(* Logix 5000 Rung export; software revision 16.04 *)

MODULES
   Local : vendor None type None code None
   GSC : vendor None type None code None
END_MODULES

TYPE GSCBLOCKSTATUS :   // This shows all blocks that were used by the module
STRUCT
   Read : INT;   // Number of blocks read by the module
   Write : INT;   // Number of blocks written by the module
   Parse : INT;   // Number of blocks parsed by the module
   Err : INT;   // Number of block transfer errors
END_STRUCT
END_TYPE

TYPE GSCCONTROL :   // Ladder send special blocks to request the module to perform the request
STRUCT
   Warmboot : BOOL;   // Performs a warm boot operation on the module (software reset).
   Coldboot : BOOL;   // Performs a cold boot operation on the module (hardware and software reset).
   ConfigDone : BOOL;   // Confirms the module received its configuration from ladder logic
END_STRUCT
END_TYPE

TYPE GSCPORTDATA :   // Individual port data
STRUCT
   ReadLength : INT;   // The length of character the port is rescieving
   ReadString : SINT[4096];   // Where received data will be displayed
   WriteLength : INT;   // The length of character the port is transmitting
   WDelay : INT;   // Number of milliseconds to wait between each character sent from the port
   WriteString : SINT[4096];   // Where sent data will be placed before it is sent
END_STRUCT
END_TYPE

TYPE GSCERRORWORD :   // Bit coded error word for configuration and overflow error for MVI56-GSC module.
STRUCT
   Cfg_type : BOOL;   // Bit 0, type field configuration error
   Cfg_Baud : BOOL;   // Bit 1, baud rate field configuration error
   Cfg_Parity : BOOL;   // Bit 2, parity field configuration error
   Cfg_DataBits : BOOL;   // Bit 3, data bit field configuration error
   Cfg_StopBits : BOOL;   // Bit 4, stop bit field configuration error
   Cfg_Handshake : BOOL;   // Bit 5, handshaking field configuration error
   Cfg_RTermcount : BOOL;   // Bit 6, receive termination character count field configuration error
   Cfg_RPacketLen : BOOL;   // Bit 7, receive packet length field configuration error
   Cfg_RTimeout : BOOL;   // Bit 8, receive message timeout field configuration error
   Cfg_RDelay : BOOL;   // Bit 9, receive intercharacter delay field configuration error
   Cfg_WTimeout : BOOL;   // Bit 10, write message timeout field configuration error
   Resv_Bit11 : BOOL;   // Bit 11
   Resv_Bit12 : BOOL;   // Bit 12
   Resv_Bit13 : BOOL;   // Bit 13
   Resv_Bit14 : BOOL;   // Bit 14
   Err_ROverflow : BOOL;   // Bit 15, receive overflow error
END_STRUCT
END_TYPE

TYPE GSCPORTSTAT :   // Port status Data
STRUCT
   RxState : INT;   // State of receive task
   RxCharCnt : INT;   // Number of characters received on port
   RxMsgCnt : INT;   // Number of messages received on port
   TxState : INT;   // State of transmit task
   TxCharCnt : INT;   // Number of characters transmitted on port
   TxMsgCnt : INT;   // Number of messages transmitted on port
   ErrorWord : GSCERRORWORD;   // Error/Configuration Word for port
END_STRUCT
END_TYPE

TYPE GSCMODULEDEF :   // This defines the complete module tags
STRUCT
   CONFIG : GSCPORTCONFIG;   // Port configuration parameters
   DATA : GSCDATA;   // Port sent and received data
   STATUS : GSCSTATUS;   // Module status data and individual port status
   CONTROL : GSCCONTROL;   // Module control parameters
   UTIL : GSCUTIL;   // Tags used by the module
END_STRUCT
END_TYPE

TYPE GSCUTIL :   // Used by the module for block hand shaking
STRUCT
   LastRead : SINT;   // This is used to read the input image from the processor
   LastWrite : SINT;   // This is used to write the output image to the processor
   BackplaneFail : INT;   // This is used to control number of backplane failures before module stops communicating on both gsc ports
   P1WriteLast : INT;   // Port 1 last write data in the array
   P2Writelast : INT;   // Port 2 last data in the array
   P1ArrayIndex : INT;   // This is the index reference within the read or write data array for port1
   P2ArrayIndex : INT;   // This is the index reference within the read or write data array for port 2
   P1RSindex : INT;   // used when more than 200 characters are received on the port 1
   P2RSindex : INT;   // used when more than 200 characters are received on the port 2
   P1Temp1 : INT;   // This temp parameter for port 1 is used to copy SINT to an INT in order to read a vlaue is higher than 127 characters
   P2Temp2 : INT;   // This temp parameter for port 2 is used to copy SINT to an INT in order to read a vlaue is higher than 127 characters
   Scratch1 : INT;   // Used to calculate number of characters read by the port
   Scratch2 : INT;   // Used to calculate number of characters read by the port
END_STRUCT
END_TYPE

TYPE GSCDATA :   // The following contains the data read in on the port and to be written out the port.
STRUCT
   Port1 : GSCPORTDATA;   // Port 1 data
   Port2 : GSCPORTDATA;   // Port 2 data
END_STRUCT
END_TYPE

TYPE GSCPORTCONFIG :   // Shows both ports configuration
STRUCT
   Port1 : GSCPORTCONFIGPARA;   // Port 1 configuration data
   Port2 : GSCPORTCONFIGPARA;   // Port 2 configuration data
END_STRUCT
END_TYPE

TYPE GSCSTATUS :   // Module Status data
STRUCT
   PassCnt : INT;   // Program cycle counter for module
   Product : INT[2];   // Product code for module (GSC)
   Rev : INT[2];   // Revision level of module's code
   OP : INT[2];   // Operating system version for module
   Run : INT[2];   // Run number for module
   BlockStatus : GSCBLOCKSTATUS;   // Data block transfer statistics
   Port1 : GSCPORTSTAT;   // Status for port1
   Port2 : GSCPORTSTAT;   // Status for port 2
END_STRUCT
END_TYPE

TYPE GSCPORTCONFIGPARA :   // The following are the configuration parameters for the port of the MVI56-GSC module.
STRUCT
   Enabled : INT;   // 0=Disable port, 1=Enable port
   Type : INT;   // Type of control used to flush data received on port
   Baudrate : INT;   // Baud rate for communications
   Parity : INT;   // Parity (0=none, 1=odd, 2=even, 3=mark, 4=space)
   DataBits : INT;   // Data bits (5, 6, 7, or 8)
   StopBits : INT;   // Stop bits (1 or 2)
   RTSOn : INT;   // RTS delay before sending data
   RTSOff : INT;   // RTS delay after sending message
   Handshaking : INT;   // Type of Handshaking (0=none, 1=RTSCTS, 2=DTRDSR,3=XONXOFF)
   RTermCnt : INT;   // Number of termination characters for received message for control
   RTermChar : SINT[12];   // Characters for termination control
   RPacketLen : INT;   // Fixed packet length value
   RTimeout : INT;   // Message timeout value for control
   RDelay : INT;   // Intercharacter timeout for control
   WTermCnt : INT;   // Not used
   WTermChar : SINT[12];   // Not used
   WPacketLen : INT;   // Not used
   WTimeout : INT;   // Timeout for sending a message out the port
   Spare : INT;   // Not used
   WMinDelay : INT;   // Minimum delay before transmitting message out port
END_STRUCT
END_TYPE

ADD_ON_INSTRUCTION AOI56GSC   (* revision 1.9, vendor ProSoft Technology Inc., ExecutePrescan *)
// Add-On For MVI56GSC and MVI56EGSC Modules.
// Revision note:
// 7/6/17
// Minor fix to FLL instruction
// 6/7/16
// Confirmed fix regarding 'Copy' length on the GSC.UTIL.PxTempx
// Help:
// 05/09/13
// AOI was fixed so that GSC.UTIL.Backplane.Fail parameter was affecting the intercharacter delay parameter in the module
VAR_IN_OUT
   Connection_Input : SINT[500]; {required}
   Connection_Output : SINT[496]; {required}
   GSC : GSCMODULEDEF; {required}
END_VAR
VAR
   MJFAULTS : DINT[12];
   ONS_Config : BOOL;
END_VAR

ROUTINE Logic   (* ladder *)
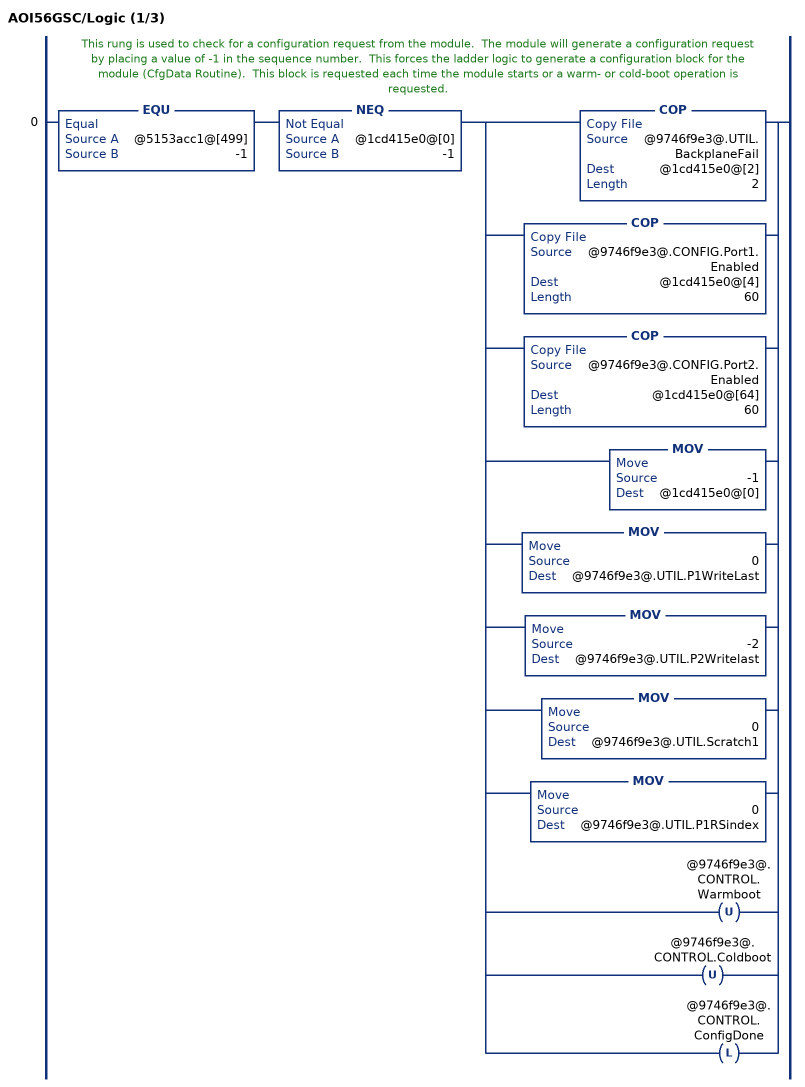
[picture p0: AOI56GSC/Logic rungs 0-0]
   // This rung is used to check for a configuration request from the module.  The module will generate a configuration request by placing a value of -1 in the sequence number.  This forces the ladder logic to generate a configuration block for the module (CfgData Routine).  This block is requested each time the module starts or a warm- or cold-boot operation is requested.
   0: EQU(@5153acc1@[499],-1)NEQ(@1cd415e0@[0],-1)[COP(@9746f9e3@.UTIL.BackplaneFail,@1cd415e0@[2],2) ,COP(@9746f9e3@.CONFIG.Port1.Enabled,@1cd415e0@[4],60) ,COP(@9746f9e3@.CONFIG.Port2.Enabled,@1cd415e0@[64],60) ,MOV(-1,@1cd415e0@[0]) ,MOV(0,@9746f9e3@.UTIL.P1WriteLast) ,MOV(-2,@9746f9e3@.UTIL.P2Writelast) ,MOV(0,@9746f9e3@.UTIL.Scratch1) ,MOV(0,@9746f9e3@.UTIL.P1RSindex) ,OTU(@9746f9e3@.CONTROL.Warmboot) ,OTU(@9746f9e3@.CONTROL.Coldboot) ,OTL(@9746f9e3@.CONTROL.ConfigDone) ];
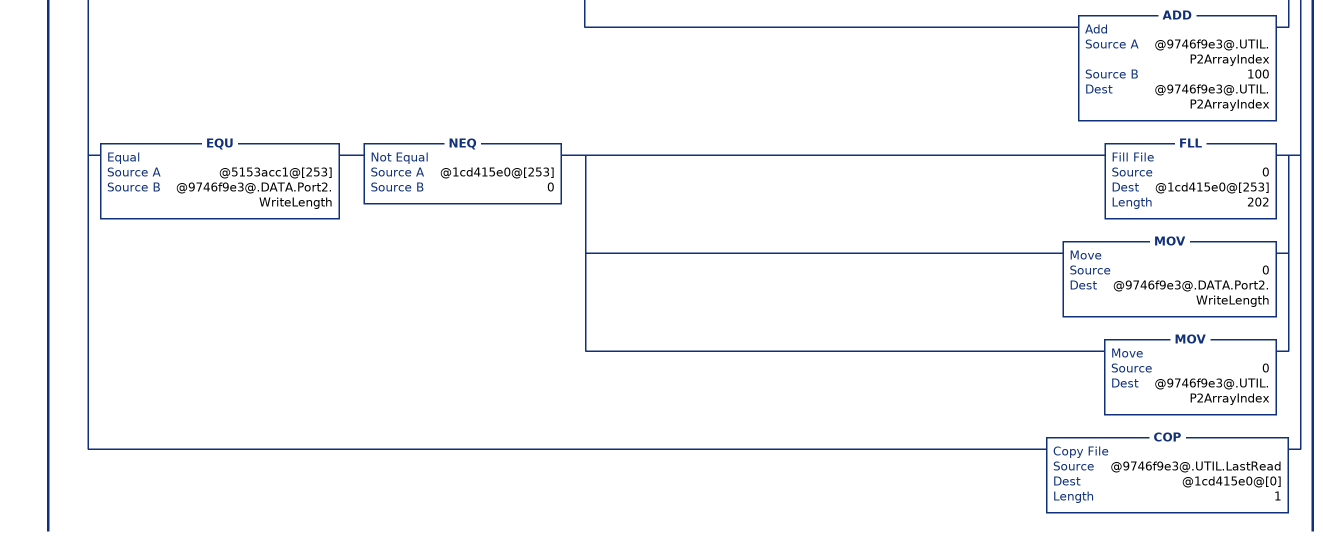
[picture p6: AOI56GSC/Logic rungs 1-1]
   // This rung is executed when a new data block is received from the module.  These blocks will have a sequence number range of 0 to 127.  When a new block is received, the ProcessBlock routine is executed to handle the newly received data.
   1: NEQ(@5153acc1@[499],@9746f9e3@.UTIL.LastRead)NEQ(@5153acc1@[499],-1)XIO(@9746f9e3@.CONTROL.Warmboot)XIO(@9746f9e3@.CONTROL.Coldboot)[COP(@5153acc1@[499],@9746f9e3@.UTIL.LastRead,1) ,GEQ(@9746f9e3@.UTIL.LastRead,0) [COP(@5153acc1@[210],@9746f9e3@.STATUS.PassCnt,1) ,COP(@5153acc1@[1],@9746f9e3@.UTIL.P1Temp1,1) ,COP(@5153acc1@[251],@9746f9e3@.UTIL.P2Temp2,1) ,COP(@5153acc1@[212],@9746f9e3@.STATUS.Product[0],8) ,COP(@5153acc1@[228],@9746f9e3@.STATUS.BlockStatus.Read,4) ,COP(@5153acc1@[236],@9746f9e3@.STATUS.Port1.RxState,6) ,COP(@5153acc1@[248],@9746f9e3@.STATUS.Port1.ErrorWord,1) ,COP(@5153acc1@[456],@9746f9e3@.STATUS.Port2.RxState,6) ,COP(@5153acc1@[468],@9746f9e3@.STATUS.Port2.ErrorWord,1) ,EQU(@9746f9e3@.UTIL.P1Temp1,-1) LES(@9746f9e3@.UTIL.P1RSindex,20) [COP(@5153acc1@[5],@9746f9e3@.DATA.Port1.ReadString[@9746f9e3@.UTIL.P1RSindex*200],200) ,ADD(1,@9746f9e3@.UTIL.P1RSindex,@9746f9e3@.UTIL.P1RSindex) ,MUL(@9746f9e3@.UTIL.P1RSindex,200,@9746f9e3@.UTIL.Scratch1) ] ,GRT(@9746f9e3@.UTIL.P1Temp1,0) [MOV(0,@9746f9e3@.DATA.Port1.ReadLength) ,COP(@5153acc1@[5],@9746f9e3@.DATA.Port1.ReadString[@9746f9e3@.UTIL.P1RSindex*200],200) ,ADD(@9746f9e3@.UTIL.P1Temp1,@9746f9e3@.UTIL.Scratch1,@9746f9e3@.DATA.Port1.ReadLength) ,MOV(0,@9746f9e3@.UTIL.P1RSindex) ,MOV(0,@9746f9e3@.UTIL.Scratch1) ] ,EQU(@9746f9e3@.UTIL.P2Temp2,-1) LES(@9746f9e3@.UTIL.P2RSindex,20) [COP(@5153acc1@[255],@9746f9e3@.DATA.Port2.ReadString[@9746f9e3@.UTIL.P2RSindex*200],200) ,ADD(1,@9746f9e3@.UTIL.P2RSindex,@9746f9e3@.UTIL.P2RSindex) ,MUL(@9746f9e3@.UTIL.P2RSindex,200,@9746f9e3@.UTIL.Scratch2) ] ,GRT(@9746f9e3@.UTIL.P2Temp2,0) [MOV(0,@9746f9e3@.DATA.Port2.ReadLength) ,COP(@5153acc1@[255],@9746f9e3@.DATA.Port2.ReadString[@9746f9e3@.UTIL.P2RSindex*200],200) ,ADD(@9746f9e3@.UTIL.P2Temp2,@9746f9e3@.UTIL.Scratch2,@9746f9e3@.DATA.Port2.ReadLength) ,MOV(0,@9746f9e3@.UTIL.P2RSindex) ,MOV(0,@9746f9e3@.UTIL.Scratch2) ] ] ,XIC(@9746f9e3@.CONTROL.ConfigDone) [FLL(0,@1cd415e0@[1],495) ,OTU(@9746f9e3@.CONTROL.ConfigDone) ] ,GRT(@9746f9e3@.DATA.Port1.WriteLength,100) LEQ(@9746f9e3@.DATA.Port1.WriteLength,4096) [COP(@9746f9e3@.DATA.Port1.WriteString[@9746f9e3@.UTIL.P1ArrayIndex],@1cd415e0@[5],100) ,MOV(100,@1cd415e0@[3]) ] ,GRT(@9746f9e3@.DATA.Port1.WriteLength,0) LEQ(@9746f9e3@.DATA.Port1.WriteLength,100) [COP(@9746f9e3@.DATA.Port1.WriteString[@9746f9e3@.UTIL.P1ArrayIndex],@1cd415e0@[5],@9746f9e3@.DATA.Port1.WriteLength) ,COP(@9746f9e3@.DATA.Port1.WDelay,@1cd415e0@[1],2) ,MOV(@9746f9e3@.DATA.Port1.WriteLength,@1cd415e0@[3]) ] ,NEQ(@5153acc1@[3],@9746f9e3@.DATA.Port1.WriteLength) GRT(@5153acc1@[3],0) [FLL(0,@1cd415e0@[3],202) ,SUB(@9746f9e3@.DATA.Port1.WriteLength,100,@9746f9e3@.DATA.Port1.WriteLength) ,ADD(@9746f9e3@.UTIL.P1ArrayIndex,100,@9746f9e3@.UTIL.P1ArrayIndex) ] ,EQU(@5153acc1@[3],@9746f9e3@.DATA.Port1.WriteLength) NEQ(@1cd415e0@[3],0) [FLL(0,@1cd415e0@[3],202) ,MOV(0,@9746f9e3@.DATA.Port1.WriteLength) ,MOV(0,@9746f9e3@.UTIL.P1ArrayIndex) ] ,GRT(@9746f9e3@.DATA.Port2.WriteLength,100) LEQ(@9746f9e3@.DATA.Port2.WriteLength,4096) [COP(@9746f9e3@.DATA.Port2.WriteString[@9746f9e3@.UTIL.P2ArrayIndex],@1cd415e0@[255],100) ,MOV(100,@1cd415e0@[253]) ] ,GRT(@9746f9e3@.DATA.Port2.WriteLength,0) LEQ(@9746f9e3@.DATA.Port2.WriteLength,100) [COP(@9746f9e3@.DATA.Port2.WriteString[@9746f9e3@.UTIL.P2ArrayIndex],@1cd415e0@[255],@9746f9e3@.DATA.Port2.WriteLength) ,COP(@9746f9e3@.DATA.Port2.WDelay,@1cd415e0@[251],2) ,MOV(@9746f9e3@.DATA.Port2.WriteLength,@1cd415e0@[253]) ] ,NEQ(@5153acc1@[253],@9746f9e3@.DATA.Port2.WriteLength) GRT(@5153acc1@[253],0) [FLL(0,@1cd415e0@[253],202) ,SUB(@9746f9e3@.DATA.Port2.WriteLength,100,@9746f9e3@.DATA.Port2.WriteLength) ,ADD(@9746f9e3@.UTIL.P2ArrayIndex,100,@9746f9e3@.UTIL.P2ArrayIndex) ] ,EQU(@5153acc1@[253],@9746f9e3@.DATA.Port2.WriteLength) NEQ(@1cd415e0@[253],0) [FLL(0,@1cd415e0@[253],202) ,MOV(0,@9746f9e3@.DATA.Port2.WriteLength) ,MOV(0,@9746f9e3@.UTIL.P2ArrayIndex) ] ,COP(@9746f9e3@.UTIL.LastRead,@1cd415e0@[0],1) ];
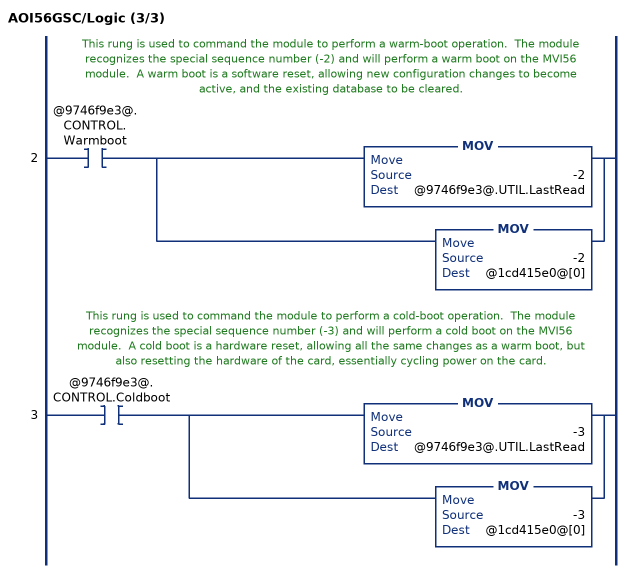
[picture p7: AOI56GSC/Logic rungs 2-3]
   // This rung is used to command the module to perform a warm-boot operation.  The module recognizes the special sequence number (-2) and will perform a warm boot on the MVI56 module.  A warm boot is a software reset, allowing new configuration changes to become active, and the existing database to be cleared.
   2: XIC(@9746f9e3@.CONTROL.Warmboot)[MOV(-2,@9746f9e3@.UTIL.LastRead) ,MOV(-2,@1cd415e0@[0]) ];
   // This rung is used to command the module to perform a cold-boot operation.  The module recognizes the special sequence number (-3) and will perform a cold boot on the MVI56 module.  A cold boot is a hardware reset, allowing all the same changes as a warm boot, but also resetting the hardware of the card, essentially cycling power on the card.
   3: XIC(@9746f9e3@.CONTROL.Coldboot)[MOV(-3,@9746f9e3@.UTIL.LastRead) ,MOV(-3,@1cd415e0@[0]) ];
END_ROUTINE

ROUTINE Prescan   (* ladder *)
// PowerUp
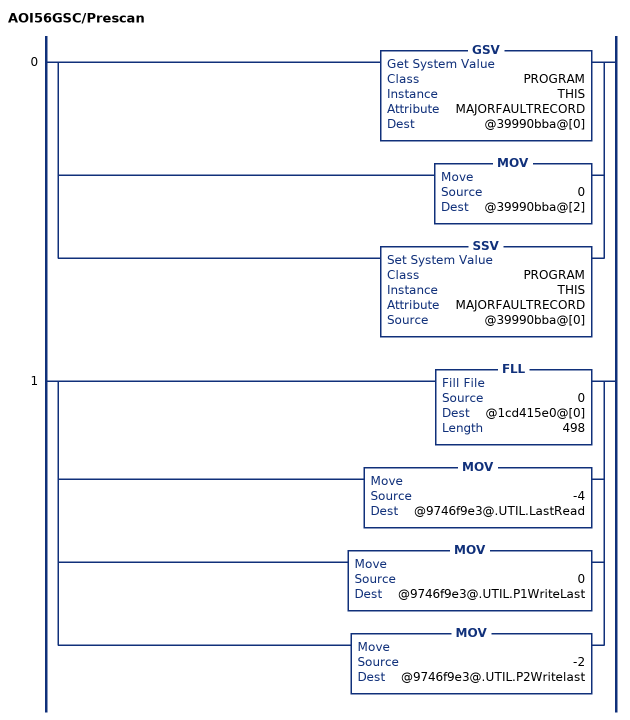
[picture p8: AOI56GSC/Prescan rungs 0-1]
   0: [GSV(PROGRAM,THIS,MAJORFAULTRECORD,@39990bba@[0]) ,MOV(0,@39990bba@[2]) ,SSV(PROGRAM,THIS,MAJORFAULTRECORD,@39990bba@[0]) ];
   1: [FLL(0,@1cd415e0@[0],498) ,MOV(-4,@9746f9e3@.UTIL.LastRead) ,MOV(0,@9746f9e3@.UTIL.P1WriteLast) ,MOV(-2,@9746f9e3@.UTIL.P2Writelast) ];
END_ROUTINE
END_ADD_ON_INSTRUCTION

VAR_GLOBAL   (* controller tags *)
   GSC : GSCMODULEDEF;
   AOI56GSC : AOI56GSC;
   Local:1:I : PS:MVI56E_GSC:I:0;
   Local:1:O : PS:MVI56E_GSC:O:0;
END_VAR

PROGRAM MainProgram

ROUTINE MainRoutine   (* ladder *)
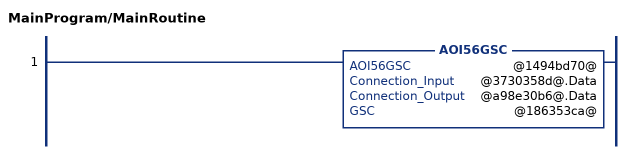
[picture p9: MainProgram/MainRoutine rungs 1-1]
   1: AOI56GSC(@1494bd70@,@3730358d@.Data,@a98e30b6@.Data,@186353ca@);
END_ROUTINE
END_PROGRAM
